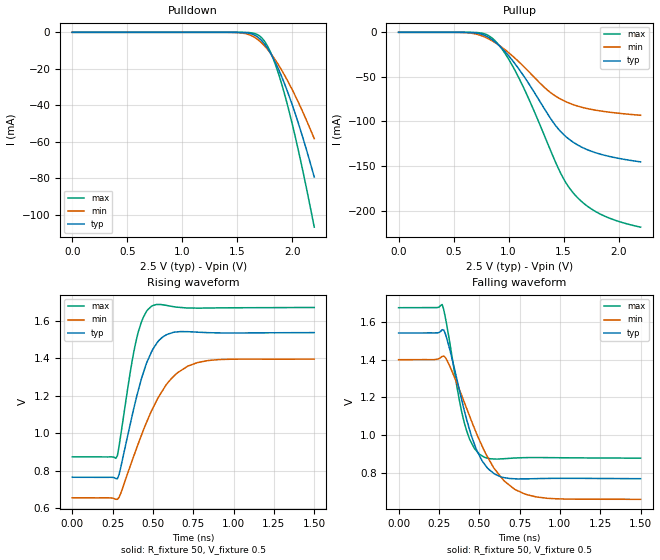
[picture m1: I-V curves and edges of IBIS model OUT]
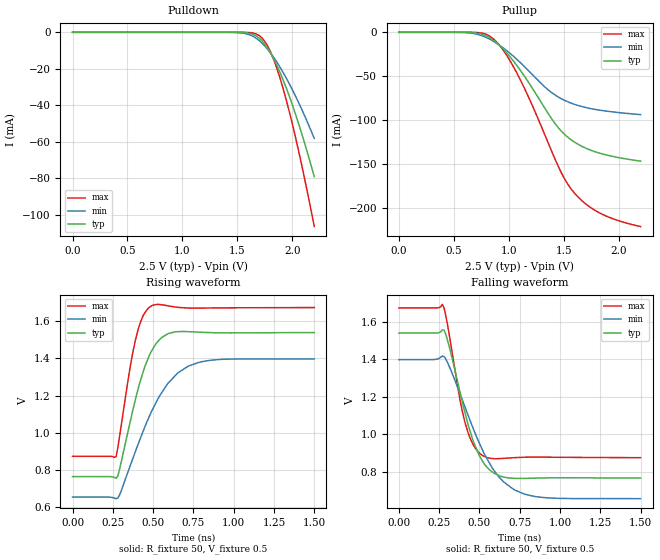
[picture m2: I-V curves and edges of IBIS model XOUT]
|   IBIS File sg7050een_25v.ibs
[IBIS Ver]   3.2
[File name]   sg7050een_25v.ibs
[File Rev]   1.0
[Date]   2016/08/17 11:07:03
[Source]
[Disclaimer]
Seiko Epson Corporation makes no warranty with respect to the information
contained herein.
[Copyright]
Copyright(C) 2016, Seiko Epson Corporation. All rights reserved.
|   Component SG7050EEN 2.5V
[Component]   sg7050een_25v
[Manufacturer]   Seiko Epson Corporation
[Package]
R_pkg   0.036   NA   NA
L_pkg   4.00n   NA   NA
C_pkg   0.70p   NA   NA
[Pin] signal_name   model_name   R_pin   L_pin   C_pin
1   OE   NC
2   NC   NC
3   GND   GND
4   OUT   OUT   0.043   4.00n   0.90p
5   XOUT   XOUT   0.028   4.00n   0.51p
6   VCC   POWER
[Diff Pin] inv_pin vdiff   tdelay_typ
4   5   0   0
| Models and submodels in the file (2): OUT (Output_ECL), XOUT (Output_ECL)
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[Model]   OUT
Model_type Output_ECL
Enable Active-High
Polarity Non-Inverting
Vref=0.5
Vmeas=1.17
Rref=50
Cref=0
C_comp   70f   70f   70f
[Temperature Range] 25   105   -40
[Voltage Range]   2.5   2.375   2.625
[Pullup Reference]  2.5   2.375   2.625
[Pulldown Reference]2.5   2.375   2.625
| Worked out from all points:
|   falling waveform, R_fixture 50, V_fixture 0.5: 20-80 % time 146ps typ, 235ps min, 104ps max; typ from 1.54 V to 0.768 V
|   rising waveform, R_fixture 50, V_fixture 0.5: 20-80 % time 138ps typ, 224ps min, 92.7ps max; typ from 0.765 V to 1.54 V
[Pullup]
0V        5.969pA    12.9pA     4.036pA
625mV     -108.8uA   -500uA     -13.26uA
775mV     -3.072mA   -4.808mA   -1.477mA
850mV     -8.265mA   -9.47mA    -6.432mA
950mV     -19.3mA    -17.84mA   -20.46mA
1.075V    -38.05mA   -30.96mA   -46.7mA
1.425V    -104.2mA   -71.4mA    -145.2mA
1.5V      -114.7mA   -76.64mA   -164.3mA
1.575V    -122.2mA   -80.59mA   -178.3mA
1.7V      -130.9mA   -85.14mA   -193.6mA
1.825V    -136.4mA   -88.02mA   -203.4mA
2.2V      -145.3mA   -93.07mA   -218.6mA
[Pulldown]
0V        5.173pA    17.34pA    4.15pA
1.5V      -27.76uA   -158.8uA   -2.412uA
1.625V    -767.9uA   -1.707mA   -243.1uA
1.7V      -3.252mA   -4.608mA   -1.837mA
1.75V     -6.546mA   -7.554mA   -5.024mA
1.8V      -11.17mA   -11.22mA   -10.54mA
1.85V     -16.95mA   -15.51mA   -18.17mA
1.925V    -27.44mA   -22.95mA   -32.75mA
1.975V    -35.45mA   -28.5mA    -44.12mA
2.05V     -48.78mA   -37.62mA   -63.18mA
2.125V    -63.48mA   -47.59mA   -84.19mA
2.2V      -79.31mA   -58.27mA   -106.7mA
[Falling Waveform]
R_fixture=50
V_fixture=0.5
V_fixture_min=0.375
V_fixture_max=0.625
0s        1.541V     1.399V     1.675V
270ps     1.559V     1.417V     1.693V
300ps     1.508V     1.396V     1.576V
370ps     1.264V     1.256V     1.214V
410ps     1.12V      1.167V     1.056V
470ps     950.9mV    1.035V     927.8mV
520ps     859.3mV    936.6mV    887.1mV
650ps     773.7mV    759.8mV    873.4mV
780ps     766.5mV    687mV      879.2mV
1.5ns     767.6mV    657.9mV    876.5mV
[Rising Waveform]
R_fixture=50
V_fixture=0.5
V_fixture_min=0.375
V_fixture_max=0.625
0s        765.1mV    655.4mV    874.2mV
280ps     757.5mV    647.1mV    880.8mV
360ps     1.051V     826.8mV    1.329V
400ps     1.199V     923mV      1.51V
440ps     1.322V     1.015V     1.619V
490ps     1.433V     1.117V     1.678V
540ps     1.499V     1.201V     1.688V
620ps     1.538V     1.298V     1.678V
780ps     1.54V      1.379V     1.669V
1.5ns     1.538V     1.396V     1.672V
[Ramp]
R_load=50
dV/dt_r   4.654E-1/1.394E-10   4.457E-1/2.246E-10   4.808E-1/9.333E-11
dV/dt_f   4.654E-1/1.472E-10   4.457E-1/2.361E-10   4.808E-1/1.050E-10
|[End   OUT
[Model]   XOUT
Model_type Output_ECL
Enable Active-High
Polarity Inverting
Vref=0.5
Vmeas=1.17
Rref=50
Cref=0
C_comp   70f   70f   70f
[Temperature Range] 25   105   -40
[Voltage Range]   2.5   2.375   2.625
[Pullup Reference]  2.5   2.375   2.625
[Pulldown Reference]2.5   2.375   2.625
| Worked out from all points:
|   falling waveform, R_fixture 50, V_fixture 0.5: 20-80 % time 146ps typ, 227ps min, 104ps max; typ from 1.54 V to 0.767 V
|   rising waveform, R_fixture 50, V_fixture 0.5: 20-80 % time 140ps typ, 229ps min, 93.3ps max; typ from 0.765 V to 1.54 V
[Pullup]
0V        6.878pA    10.63pA    3.809pA
625mV     -108.7uA   -499.5uA   -13.23uA
775mV     -3.069mA   -4.804mA   -1.475mA
850mV     -8.258mA   -9.464mA   -6.425mA
950mV     -19.29mA   -17.83mA   -20.44mA
1.075V    -38.03mA   -30.95mA   -46.66mA
1.2V      -60.75mA   -46.18mA   -79.23mA
1.425V    -104.5mA   -71.61mA   -145.3mA
1.575V    -122.9mA   -80.96mA   -179.4mA
1.7V      -131.8mA   -85.59mA   -195.3mA
1.825V    -137.4mA   -88.53mA   -205.4mA
2.2V      -146.6mA   -93.65mA   -221mA
[Pulldown]
0V        7.105pA    16.09pA    3.922pA
1.5V      -27.59uA   -158.2uA   -2.391uA
1.625V    -764.3uA   -1.702mA   -241.6uA
1.7V      -3.241mA   -4.597mA   -1.828mA
1.75V     -6.528mA   -7.539mA   -5.005mA
1.8V      -11.15mA   -11.2mA    -10.51mA
1.85V     -16.92mA   -15.49mA   -18.12mA
1.925V    -27.39mA   -22.92mA   -32.68mA
1.975V    -35.4mA    -28.47mA   -44.04mA
2.05V     -48.72mA   -37.58mA   -63.08mA
2.125V    -63.41mA   -47.54mA   -84.06mA
2.2V      -79.23mA   -58.22mA   -106.6mA
[Falling Waveform]
R_fixture=50
V_fixture=0.5
V_fixture_min=0.375
V_fixture_max=0.625
0s        1.541V     1.399V     1.675V
270ps     1.558V     1.418V     1.694V
300ps     1.508V     1.387V     1.594V
380ps     1.223V     1.217V     1.182V
410ps     1.117V     1.147V     1.065V
460ps     967.7mV    1.035V     946.2mV
520ps     857.1mV    914.8mV    887.1mV
650ps     773.4mV    747.2mV    872.5mV
780ps     765.7mV    681.7mV    878.6mV
1.5ns     767.3mV    657.5mV    876.3mV
[Rising Waveform]
R_fixture=50
V_fixture=0.5
V_fixture_min=0.375
V_fixture_max=0.625
0s        765mV      655.3mV    874.2mV
270ps     756.3mV    646.5mV    872.5mV
290ps     797mV      662.7mV    970.6mV
390ps     1.178V     899.3mV    1.497V
440ps     1.332V     1.013V     1.633V
490ps     1.438V     1.114V     1.681V
550ps     1.509V     1.211V     1.688V
650ps     1.543V     1.318V     1.674V
780ps     1.541V     1.377V     1.67V
1.5ns     1.538V     1.397V     1.672V
[Ramp]
R_load=50
dV/dt_r   4.653E-1/1.409E-10   4.457E-1/2.298E-10   4.806E-1/9.385E-11
dV/dt_f   4.653E-1/1.464E-10   4.457E-1/2.281E-10   4.806E-1/1.047E-10
|[End   XOUT
